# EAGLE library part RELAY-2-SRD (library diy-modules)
2-Channel Relay Module based on SRD-05VDC-SL-C relays Click here to find device on ebay.com
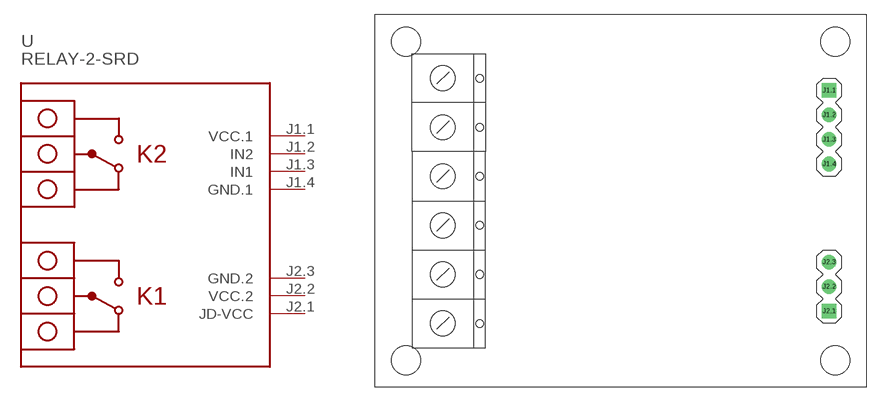
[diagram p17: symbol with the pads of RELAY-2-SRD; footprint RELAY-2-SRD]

Designator prefix -

## RELAY-2-SRD  [RELAY-2-SRD]
J1.1  VCC.1  pwr
J1.2  IN2
J1.3  IN1
J1.4  GND.1  pwr
J2.1  JD-VCC
J2.2  VCC.2  pwr
J2.3  GND.2  pwr

## Footprint RELAY-2-SRD (pad centres in mm)
2-Channel Relay Module based on SRD-05VDC-SL-C relays
drill 1 square: J1.1 21.59,11.43; J2.1 21.59,-11.43
drill 1: J1.2 21.59,8.89; J1.3 21.59,6.35; J1.4 21.59,3.81; J2.2 21.59,-8.89; J2.3 21.59,-6.35
hole 3 at -22.225,16.51
hole 3 at 22.225,16.51
hole 3 at 22.225,-16.51
hole 3 at -22.225,-16.51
